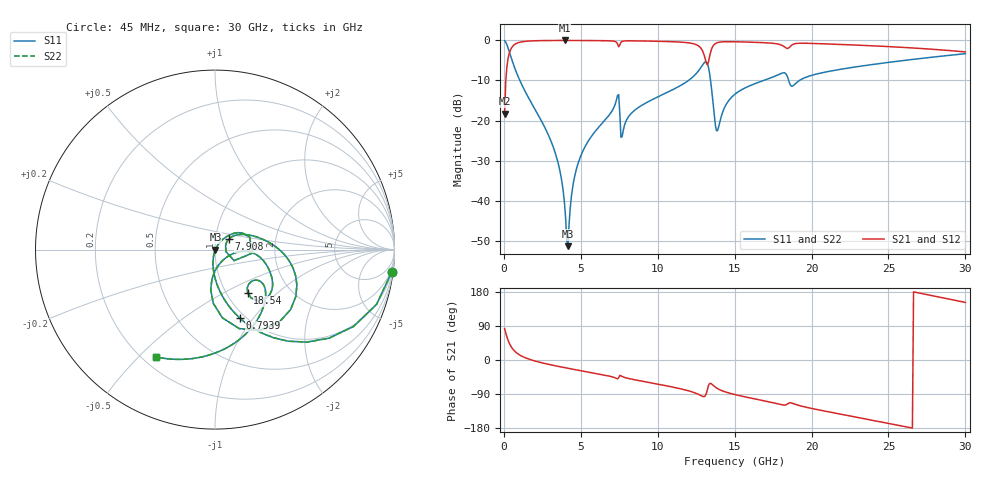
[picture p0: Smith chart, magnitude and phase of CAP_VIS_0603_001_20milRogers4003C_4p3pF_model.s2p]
! S-parameter model data by Modelithics Inc.  support@modelithics.com  813-866-6335  Tampa FL USA
! S-Parameter data specifications:
! Substrate: 20-mil Rogers 4003C, substrate thickness, H=0.508mm, Dielectric constant, Er=3.75
! PCB Mounting Pad Footprint: Pad width, PadW=0.90mm , Pad length, PadL=1.00mm , Pad gap, PadG (edge-to-edge)=1.00mm , Reference planes=3.0mm apart
! Created Wed Nov 18 13:22:43 2015
# hz S ma R 50
! 2 Port Network Data from SP1.SP block
! freq  magS11  angS11  magS21  angS21  magS12  angS12  magS22  angS22
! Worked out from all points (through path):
!   401 points, 45 MHz to 30 GHz, reference 50 ohm
!   highest |S21| = -0.02 dB at 3.939 GHz (marker M1); lowest = -18.3 dB at 45 MHz (marker M2)
!   group delay of S21, straight-line fit = 20.2 ps
!   lowest |S11| = -51.3 dB at 4.164 GHz (marker M3), VSWR 1.01, Z = 50.3 + j0.0277 ohm
!   |S11| at or under -10 dB: 1.035 GHz to 12 GHz (10.97 GHz wide, 168 % of centre); 13.43 GHz to 16.88 GHz (3.448 GHz wide, 22.8 % of centre); 18.51 GHz to 19.21 GHz (699.3 MHz wide, 3.71 % of centre)
!   |S22| runs from -51.3 to -0.1 dB; largest |S21 - S12| = 0
!   S11 on the Smith chart (normalised r, x): 45 MHz: 1, -16; 793.9 MHz: 0.94, -0.86; 7.908 GHz: 1.16, +0.13; 18.54 GHz: 1.25, -0.67; 30 GHz: 0.25, -0.56
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4.5e7  0.9926 -7.2  0.1216 82.8  0.1216 82.8  0.9926 -7.2
3.4455e8  0.7267 -45.2  0.6864 44.8  0.6864 44.8  0.7267 -45.2
7.93875e8  0.4072 -70.0  0.9123 19.9  0.9123 19.9  0.4072 -70.0
3.190275e9  0.04776 -101.5  0.9965 -14.0  0.9965 -14.0  0.04776 -101.5
3.93915e9  0.009289 -95.6  0.9973 -20.1  0.9973 -20.1  0.009289 -95.6
4.163812e9  0.00272 5.8  0.9972 -21.9  0.9972 -21.9  0.00272 5.8
4.53825e9  0.01763 57.0  0.9969 -24.7  0.9969 -24.7  0.01763 57.0
5.062462e9  0.03891 57.3  0.9961 -28.7  0.9961 -28.7  0.03891 57.3
7.309088e9  0.179 30.9  0.9503 -48.3  0.9503 -48.3  0.179 30.9
7.683525e9  0.06289 20.3  0.9699 -43.4  0.9699 -43.4  0.06289 20.3
7.908188e9  0.0956 37.2  0.9848 -46.8  0.9848 -46.8  0.0956 37.2
1.007992e10  0.2009 24.2  0.9734 -64.3  0.9734 -64.3  0.2009 24.2
1.240144e10  0.3677 -1.3  0.8982 -86.5  0.8982 -86.5  0.3677 -1.3
1.292565e10  0.4971 -23.4  0.7312 -96.1  0.7312 -96.1  0.4971 -23.4
1.32252e10  0.516 -60.6  0.4949 -78.4  0.4949 -78.4  0.516 -60.6
1.352475e10  0.2241 -96.1  0.8017 -64.1  0.8017 -64.1  0.2241 -96.1
1.389919e10  0.07595 -36.3  0.9389 -75.7  0.9389 -75.7  0.07595 -36.3
1.50225e10  0.2136 -5.2  0.961 -91.3  0.961 -91.3  0.2136 -5.2
1.854221e10  0.3033 -53.1  0.813 -113.5  0.813 -113.5  0.3033 -53.1
2.003996e10  0.368 -40.0  0.9158 -128.1  0.9158 -128.1  0.368 -40.0
2.505742e10  0.5332 -78.5  0.8353 -167.7  0.8353 -167.7  0.5332 -78.5
3e10  0.6825 -118.8  0.718 151.9  0.718 151.9  0.6825 -118.8
